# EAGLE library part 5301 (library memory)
MEMORY
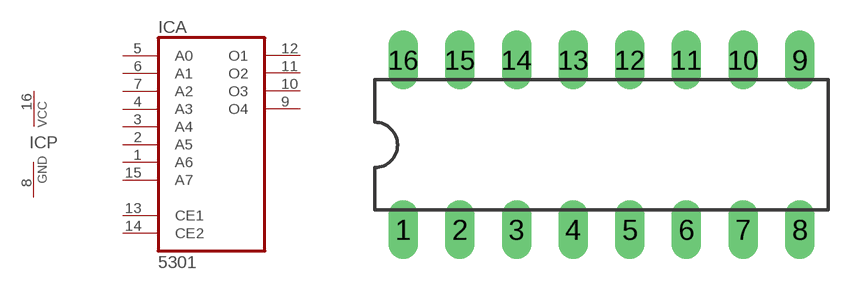
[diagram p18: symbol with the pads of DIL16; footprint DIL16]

Designator prefix IC; gates A=5301 P=PWRN

## 5301  [DIL16]
1  A:A6  in
2  A:A5  in
3  A:A4  in
4  A:A3  in
5  A:A0  in
6  A:A1  in
7  A:A2  in
8  P:GND  pwr
9  A:O4  hiz
10  A:O3  hiz
11  A:O2  hiz
12  A:O1  hiz
13  A:CE1  in
14  A:CE2  in
15  A:A7  in
16  P:VCC  pwr

## Footprint DIL16 (pad centres in mm)
Dual In Line Package
drill 0.813 long: 1 -8.89,-3.81; 2 -6.35,-3.81; 3 -3.81,-3.81; 4 -1.27,-3.81; 5 1.27,-3.81; 6 3.81,-3.81; 7 6.35,-3.81; 8 8.89,-3.81; 9 8.89,3.81; 10 6.35,3.81; 11 3.81,3.81; 12 1.27,3.81; 13 -1.27,3.81; 14 -3.81,3.81; 15 -6.35,3.81; 16 -8.89,3.81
